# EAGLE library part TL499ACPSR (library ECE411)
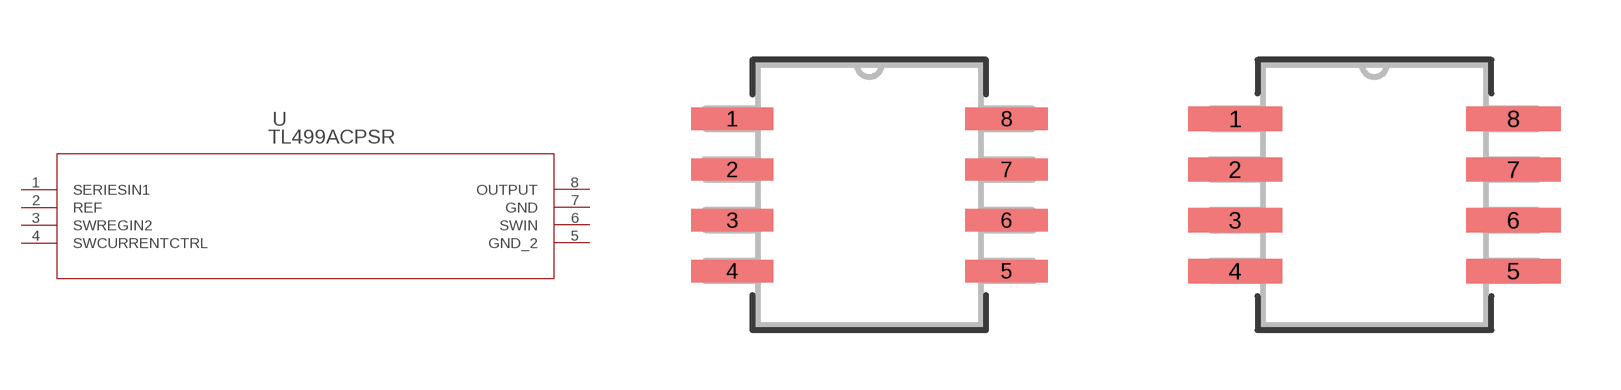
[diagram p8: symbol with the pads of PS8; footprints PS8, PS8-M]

Designator prefix U

## TL499ACPSR (MANUFACTURER_PART_NUMBER: TL499ACPSR; VENDOR: Texas Instruments)  [PS8]
1  SERIESIN1  in
2  REF  pas
3  SWREGIN2  in
4  SWCURRENTCTRL  pas
5  GND_2  pwr
6  SWIN  in
7  GND  pwr
8  OUTPUT  out

## TL499ACPSRPS8-M (MANUFACTURER_PART_NUMBER: TL499ACPSR; VENDOR: Texas Instruments)  [PS8-M]
Pads as for PS8

## TL499ACPSRPS8-L (MANUFACTURER_PART_NUMBER: TL499ACPSR; VENDOR: Texas Instruments)  [PS8-L]
Pads as for PS8

## Footprint PS8 (pad centres in mm)
smd 2.057 x 0.559: 1 -3.429,1.905; 2 -3.429,0.635; 3 -3.429,-0.635; 4 -3.429,-1.905; 5 3.429,-1.905; 6 3.429,-0.635; 7 3.429,0.635; 8 3.429,1.905

## Footprint PS8-M (pad centres in mm)
smd 2.362 x 0.61: 1 -3.48,1.905; 2 -3.48,0.635; 3 -3.48,-0.635; 4 -3.48,-1.905; 5 3.48,-1.905; 6 3.48,-0.635; 7 3.48,0.635; 8 3.48,1.905

## Footprint PS8-L (pad centres in mm)
smd 1.753 x 0.508: 1 -3.378,1.905; 2 -3.378,0.635; 3 -3.378,-0.635; 4 -3.378,-1.905; 5 3.378,-1.905; 6 3.378,-0.635; 7 3.378,0.635; 8 3.378,1.905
